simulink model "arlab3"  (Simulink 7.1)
settings: Solver=ode45  SolverMode=SingleTasking  StartTime=0.0  StopTime=inf  RelTol=1e-3  AbsTol=1e-6
PostLoadFcn:
  | arlab3_postloadfcn
StartFcn:
  | arlab3_startfcn
StopFcn:
  | arlab3_stopfcn
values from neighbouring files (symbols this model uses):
  h = findobj(gcf,'Type','axes')    [suptitle.m]    (also in arlab3_postloadfcn.m = 0.1)
  y = u(2)    [reg.m]    (also in sevalmode.m)
undefined symbols (not defined in the file or in its folder): w

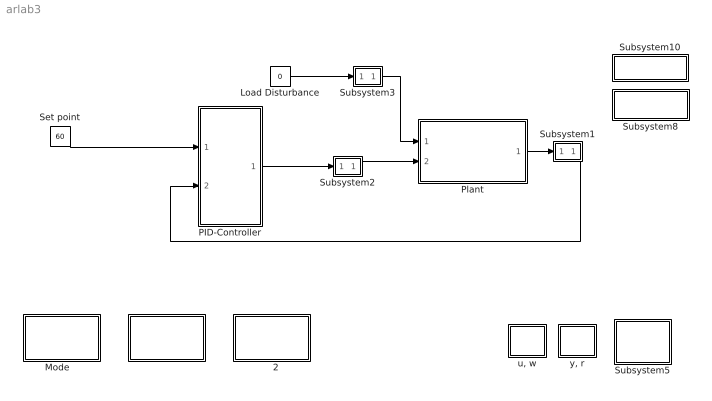
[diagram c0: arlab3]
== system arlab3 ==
  "    " : Subsystem
  "   2" : Subsystem
  Load Disturbance : Constant  Value=0
  "Mode   " : Subsystem
  PID-Controller : Subsystem
  Plant : Subsystem
  Set point : Constant  Value=60
  Subsystem1 : Subsystem  mask{vname=y}
      mask prompts: vname "Variable name"
      mask init:
      | parent = get_param(gcb,'Parent');
      | name = get_param(gcb,'Name');
      | set_param([parent '/' name '/Goto'],'GotoTag',vname)
  Subsystem10 : Subsystem
  Subsystem2 : Subsystem  mask{vname=u}
      mask prompts: vname "Variable name"
      mask init:
      | parent = get_param(gcb,'Parent');
      | name = get_param(gcb,'Name');
      | set_param([parent '/' name '/Goto'],'GotoTag',vname)
  Subsystem3 : Subsystem  mask{vname=w}
      mask prompts: vname "Variable name"
      mask init:
      | parent = get_param(gcb,'Parent');
      | name = get_param(gcb,'Name');
      | set_param([parent '/' name '/Goto'],'GotoTag',vname)
  Subsystem5 : Subsystem
  Subsystem8 : Subsystem
  "u, w" : Subsystem
  "y, r" : Subsystem
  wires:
  Set point/1 -> PID-Controller/1(In1)
  Load Disturbance/1 -> Subsystem3/1(In)
  PID-Controller/1(Out2) -> Subsystem2/1(In)
  Plant/1(Out1) -> Subsystem1/1(In)
  Subsystem1/1(Out) -> PID-Controller/2(In2)
  Subsystem2/1(Out) -> Plant/2(In2)
  Subsystem3/1(Out) -> Plant/1(In1)

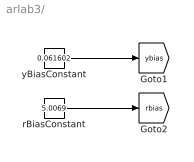
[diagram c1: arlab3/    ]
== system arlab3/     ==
  rBiasConstant : Constant  Value=5.0069
  yBiasConstant : Constant  Value=0.061602
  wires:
  yBiasConstant/1 -> [ybias]
  rBiasConstant/1 -> [rbias]

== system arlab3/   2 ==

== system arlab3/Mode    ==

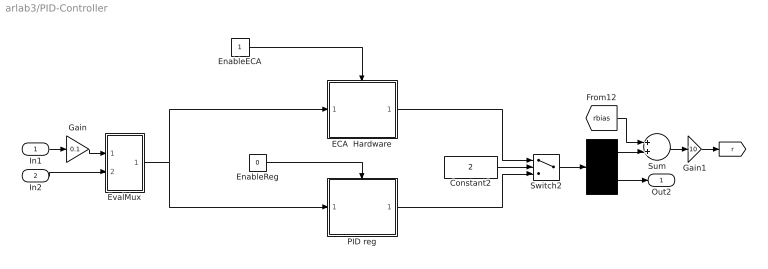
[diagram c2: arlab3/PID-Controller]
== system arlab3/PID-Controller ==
  In1 : Inport
  In2 : Inport  Port=2
  " " : Demux  Outputs=2
  Constant2 : Constant  Value=2
  ECA  Hardware : Subsystem
  EnableECA : Constant
  EnableReg : Constant  Value=0
  EvalMux : Subsystem
  Gain : Gain  Gain=0.1
  Gain1 : Gain  Gain=10
  PID reg : Subsystem
  Sum : Sum
  Switch2 : Switch  Threshold=2
  Out2 : Outport
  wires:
  Constant2/1 -> Switch2/2
  ECA  Hardware/1("[ r  u ]") -> Switch2/1
  PID reg/1("[ r u ]") -> Switch2/3
  Switch2/1 -> " "/1
  " "/2 -> Out2/1
  " "/1 -> Sum/2
  [rbias] -> Sum/1
  EnableECA/1 -> ECA  Hardware/Enable
  EnableReg/1 -> PID reg/Enable
  In2/1 -> EvalMux/2(In2)
  EvalMux/1(Out1) -> ECA  Hardware/1("[ r  y ]"), PID reg/1("[ r y ]")
  In1/1 -> Gain/1
  Gain/1 -> EvalMux/1(In1)
  Sum/1 -> Gain1/1
  Gain1/1 -> [r]

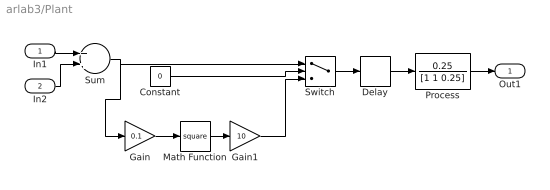
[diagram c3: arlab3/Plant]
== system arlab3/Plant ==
  In1 : Inport
  In2 : Inport  Port=2
  Constant : Constant  Value=0
  Delay : TransportDelay  DelayTime=4
  Gain : Gain  Gain=0.1
  Gain1 : Gain  Gain=10
  Math Function : Math  Operator=square
  Process : TransferFcn  Numerator=0.25  Denominator=[1 1 0.25]
  Sum : Sum
  Switch : Switch  Threshold=1
  Out1 : Outport
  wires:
  In1/1 -> Sum/1
  In2/1 -> Sum/2
  Gain/1 -> Math Function/1
  Math Function/1 -> Gain1/1
  Sum/1 -> Switch/1, Gain/1
  Switch/1 -> Delay/1
  Process/1 -> Out1/1
  Delay/1 -> Process/1
  Constant/1 -> Switch/2
  Gain1/1 -> Switch/3

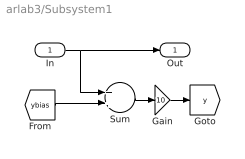
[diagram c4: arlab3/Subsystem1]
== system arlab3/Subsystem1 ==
  In : Inport
  Gain : Gain  Gain=10
  Sum : Sum
  Out : Outport
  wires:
  In/1 -> Out/1, Sum/1
  [ybias] -> Sum/2
  Sum/1 -> Gain/1
  Gain/1 -> [y]

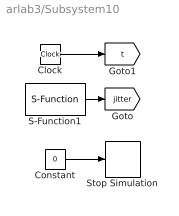
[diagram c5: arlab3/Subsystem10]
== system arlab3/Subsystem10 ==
  Clock : Clock
  Constant : Constant  Value=0
  S-Function1 : S-Function  FunctionName=realtimer  Parameters=h  EnableBusSupport=off
  Stop Simulation : Stop
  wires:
  Clock/1 -> [t]
  S-Function1/1 -> [jitter]
  Constant/1 -> Stop Simulation/1

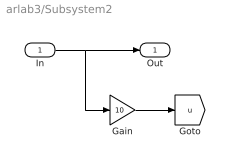
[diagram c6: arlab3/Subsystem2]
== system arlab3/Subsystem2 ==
  In : Inport
  Gain : Gain  Gain=10
  Out : Outport
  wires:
  In/1 -> Out/1, Gain/1
  Gain/1 -> [u]

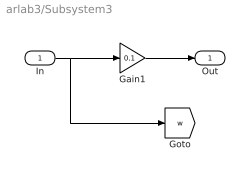
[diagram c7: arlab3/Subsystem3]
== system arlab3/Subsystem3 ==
  In : Inport
  Gain1 : Gain  Gain=0.1
  Out : Outport
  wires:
  Gain1/1 -> Out/1
  In/1 -> Gain1/1, [w]

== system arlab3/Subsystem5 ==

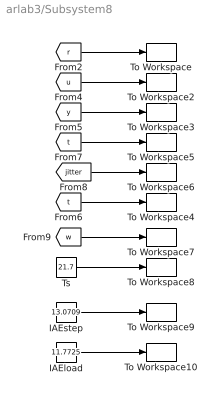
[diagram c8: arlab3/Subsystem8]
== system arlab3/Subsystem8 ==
  IAEload : Constant  Value=11.7725
  IAEstep : Constant  Value=13.0709
  To Workspace : ToWorkspace  VariableName=r  SampleTime=h  SaveFormat=Array
  To Workspace10 : ToWorkspace  VariableName=IAEload  SampleTime=h  SaveFormat=Array
  To Workspace2 : ToWorkspace  VariableName=u  SampleTime=h  SaveFormat=Array
  To Workspace3 : ToWorkspace  VariableName=y  SampleTime=h  SaveFormat=Array
  To Workspace4 : ToWorkspace  VariableName=tc  SampleTime=h  SaveFormat=Array
  To Workspace5 : ToWorkspace  VariableName=t  SampleTime=h  SaveFormat=Array
  To Workspace6 : ToWorkspace  VariableName=jitter  SampleTime=h  SaveFormat=Array
  To Workspace7 : ToWorkspace  VariableName=w  SampleTime=h  SaveFormat=Array
  To Workspace8 : ToWorkspace  VariableName=Ts  SampleTime=h  SaveFormat=Array
  To Workspace9 : ToWorkspace  VariableName=IAEstep  SampleTime=h  SaveFormat=Array
  Ts : Constant  Value=21.7
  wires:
  [t] -> To Workspace4/1
  [t] -> To Workspace5/1
  [jitter] -> To Workspace6/1
  [y] -> To Workspace3/1
  [u] -> To Workspace2/1
  [r] -> To Workspace/1
  [w] -> To Workspace7/1
  Ts/1 -> To Workspace8/1
  IAEstep/1 -> To Workspace9/1
  IAEload/1 -> To Workspace10/1

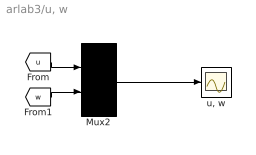
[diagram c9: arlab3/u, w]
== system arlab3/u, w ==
  Mux2 : Mux  Inputs=2
  "u, w" : Scope
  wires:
  [u] -> Mux2/1
  [w] -> Mux2/2
  Mux2/1 -> "u, w"/1

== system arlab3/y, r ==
  Mux2 : Mux  Inputs=2
  "y, r" : Scope
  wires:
  [r] -> Mux2/2
  [y] -> Mux2/1
  Mux2/1 -> "y, r"/1

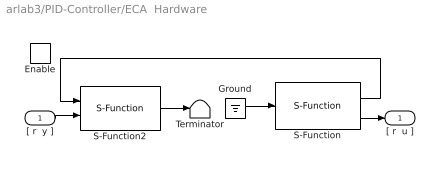
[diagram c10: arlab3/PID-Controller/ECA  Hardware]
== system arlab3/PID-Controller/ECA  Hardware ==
  "[ r  y ]" : Inport
  Enable : EnablePort
  Ground : Ground
  S-Function : S-Function  FunctionName=analogin  Parameters=h [1 0]  EnableBusSupport=off
  S-Function2 : S-Function  FunctionName=analogout  Parameters=h [1 0]  EnableBusSupport=off
  Terminator : Terminator
  "[ r  u ]" : Outport  InitialOutput=0
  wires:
  Ground/1 -> S-Function/1
  S-Function2/1 -> Terminator/1
  S-Function/1 -> S-Function2/1
  S-Function/2 -> "[ r  u ]"/1
  "[ r  y ]"/1 -> S-Function2/2

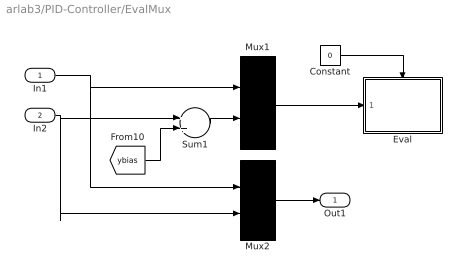
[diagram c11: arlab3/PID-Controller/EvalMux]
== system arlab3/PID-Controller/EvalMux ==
  In1 : Inport
  In2 : Inport  Port=2
  Constant : Constant  Value=0
  Eval : Subsystem
  Mux1 : Mux  Inputs=2
  Mux2 : Mux  Inputs=2
  Sum1 : Sum
  Out1 : Outport  InitialOutput=0
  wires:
  Mux2/1 -> Out1/1
  Sum1/1 -> Mux1/2
  [ybias] -> Sum1/2
  In2/1 -> Mux2/2, Sum1/1
  Mux1/1 -> Eval/1(In1)
  Constant/1 -> Eval/Enable
  In1/1 -> Mux2/1, Mux1/1

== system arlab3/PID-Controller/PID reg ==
  "[ r y ]" : Inport
  Enable : EnablePort
  S-Function : S-Function  FunctionName=reg  Parameters=h  EnableBusSupport=off
  "[ r u ]" : Outport
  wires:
  S-Function/1 -> "[ r u ]"/1
  "[ r y ]"/1 -> S-Function/1

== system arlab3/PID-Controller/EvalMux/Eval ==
  In1 : Inport
  Enable : EnablePort
  S-eval : S-Function  FunctionName=sevalmode  Parameters=h,3,4,'arlab3'  EnableBusSupport=off
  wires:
  In1/1 -> S-eval/1
